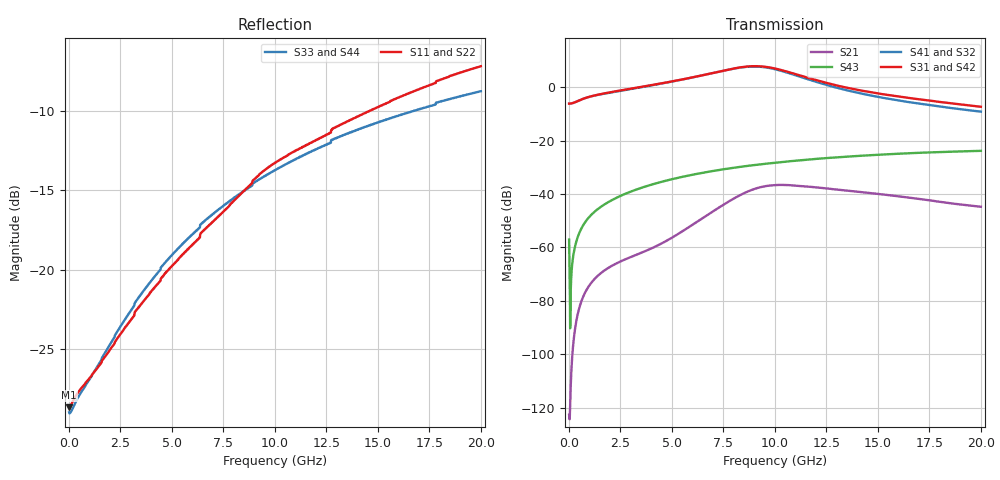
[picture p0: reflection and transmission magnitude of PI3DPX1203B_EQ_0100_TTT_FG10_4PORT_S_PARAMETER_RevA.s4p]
! NPort=4 DATA=2000 NOISE=0 GROUPDELAY=0 COMPLEX_DATAFORMAT=POLAR
! NumOfBlock=1 NumOfParam=0
! .MODEL Smodel S TSTONEFILE=PI3DPX1203B_EQ_0100_TTT_FG10_4PORT_S_PARAMETER_RevA.s4p TYPE=S
!  -- The above .MODEL line can be used for the S element in the netlist.
! The s parameter is extracted from the linear redriver, it is not bi-directional; only s(4,1)s(4,2) and s(3,1)s(3,2)
! should be the insertion loss
!Port definition:
!Port1 = input+
!Port2 = input-
!Port3 = output+
!Port4 = output-
# Hz S MA R  50
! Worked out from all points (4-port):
!   2000 points, 10 MHz to 20 GHz, reference 50 ohm
!   strongest paths, dB at 10 MHz, 5.01 GHz, 10.01 GHz, 15.01 GHz, 20 GHz:
!     S31: -6.2, 2.2, 7.0, -2.3, -7.3
!     S42: -6.2, 2.2, 7.0, -2.3, -7.3
!     S41: -6.2, 2.1, 6.7, -3.6, -9.2
!     S32: -6.2, 2.1, 6.7, -3.6, -9.1
!     S43: -57.1, -34.4, -28.3, -25.3, -23.8
!     S21: -122.7, -56.3, -36.6, -40.0, -44.8
!   lowest |S11| = -28.6 dB at 10 MHz (marker M1), VSWR 1.08, Z = 46.4 - j0.0306 ohm
!   |S11| at or under -10 dB: start of sweep to 14.61 GHz
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1e7  0.03701 -179.5  7.338e-07 10.6  0 0.0  0 0.0
     7.338e-07 10.6  0.03701 -179.5  0 0.0  0 0.0
     0.4917 -0.1  0.4917 179.9  0.03566 178.2  0.001403 -77.8
     0.4917 179.9  0.4917 -0.1  0.001403 -77.8  0.03566 178.2
1.57e9  0.05095 -144.8  0.0003342 115.1  5.114e-12 74.4  4.903e-11 115.4
        0.0003342 115.1  0.05095 -144.8  4.903e-11 115.4  5.114e-12 74.4
        0.746 4.9  0.7392 -175.1  0.05202 -142.1  0.005823 82.8
        0.7392 -175.1  0.746 4.9  0.005823 82.8  0.05202 -142.1
6.15e9  0.1224 -110.9  0.002898 139.8  1.717e-08 -115.6  1.536e-07 66.2
        0.002897 139.8  0.1224 -111.0  1.535e-07 66.2  1.717e-08 -115.6
        1.571 -46.4  1.567 135.7  0.1321 -116.9  0.02359 64.4
        1.567 135.7  1.57 -46.4  0.02359 64.4  0.1321 -116.9
8.56e9  0.1785 -105.8  0.01062 106.4  4.074e-07 157.7  1.126e-06 16.6
        0.01062 106.4  0.1785 -105.8  1.125e-06 16.6  4.073e-07 157.7
        2.418 -101.2  2.389 80.5  0.1778 -115.9  0.0332 52.0
        2.39 80.5  2.417 -101.2  0.0332 52.0  0.1778 -115.9
1.002e10  0.2172 -107.3  0.01472 63.8  1.281e-06 95.8  2.202e-06 -21.0
          0.01471 63.8  0.2172 -107.3  2.199e-06 -20.9  1.281e-06 95.8
          2.233 -148.9  2.164 32.6  0.2057 -116.3  0.03856 44.3
          2.166 32.6  2.232 -148.9  0.03856 44.3  0.2057 -116.3
1.215e10  0.2586 -108.8  0.01313 21.5  3.098e-06 30.6  3.972e-06 -48.8
          0.01313 21.5  0.2586 -108.8  3.972e-06 -48.6  3.098e-06 30.7
          1.309 166.0  1.211 -11.9  0.2416 -117.5  0.04593 33.4
          1.212 -11.9  1.308 166.1  0.04593 33.4  0.2416 -117.5
2e10  0.4361 -116.8  0.005746 -20.9  2.205e-05 -106.9  3.224e-05 -134.0
      0.005777 -21.1  0.4361 -116.8  3.232e-05 -133.9  2.207e-05 -106.9
      0.4302 82.3  0.3492 -80.9  0.3637 -123.9  0.06431 -7.1
      0.3486 -81.0  0.4307 82.3  0.06431 -7.1  0.3637 -123.9
